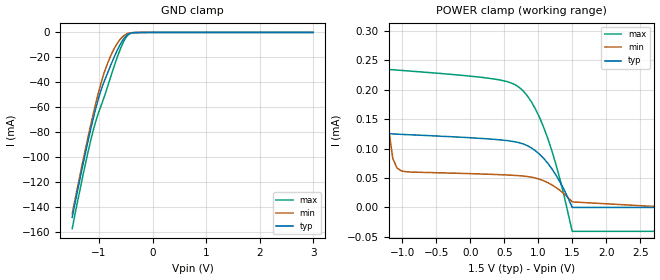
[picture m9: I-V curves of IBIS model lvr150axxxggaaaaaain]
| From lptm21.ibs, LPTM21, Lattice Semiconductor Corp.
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|   Model lvr150axxxggaaaaaain
[Model]   lvr150axxxggaaaaaain
Model_type   Input
Polarity   Non-Inverting
Enable   Active-Low
Vinl =   0.3750V
Vinh =   1.1250V
C_comp   4.2000pF   3.8000pF   7.5000pF
[Temperature Range]   25.0000   0.1050k   -40.0000
[Voltage Range]   1.5000V   1.4300V   1.5800V
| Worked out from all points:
|   GND clamp passes 1 mA (typ) near -0.43 V on its own axis
[GND_clamp]
|Voltage   I(typ)   I(min)   I(max)
-1.5V     -148.1mA   -145.3mA   -157.2mA
-1.32V    -110.1mA   -107.1mA   -118.8mA
-1.17V    -80.56mA   -77.21mA   -89.44mA
-1.05V    -59.34mA   -55.1mA    -69.88mA
-930mV    -42.38mA   -36.01mA   -55.09mA
-810mV    -29.42mA   -21.71mA   -39.47mA
-690mV    -17.27mA   -10.99mA   -23.72mA
-540mV    -5.213mA   -2.77mA    -7.437mA
-450mV    -1.326mA   -681.8uA   -1.809mA
-390mV    -401.8uA   -230.3uA   -518.8uA
-210mV    -60.72uA   -33.9uA    -106.9uA
3V        0A         0A         0A
[POWER_clamp]
|Voltage   I(typ)   I(min)   I(max)
-1.5V     579uA      4.296mA    238.7uA
-1.44V    259.3uA    2.507mA    236.9uA
-1.38V    160.3uA    1.327mA    236uA
-1.32V    134.3uA    633.5uA    235.4uA
-1.26V    127.5uA    278.5uA    234.9uA
-1.2V     125.5uA    132.8uA    234.3uA
-1.14V    124.8uA    83.11uA    233.8uA
-1.02V    124.1uA    62.34uA    232.7uA
780mV     107.8uA    53.2uA     197.7uA
1.14V     75.04uA    42.1uA     117.3uA
1.5V      -43.54nA   9.313uA    -40.74uA
3V        -43.54nA   -313.3nA   -40.74uA
